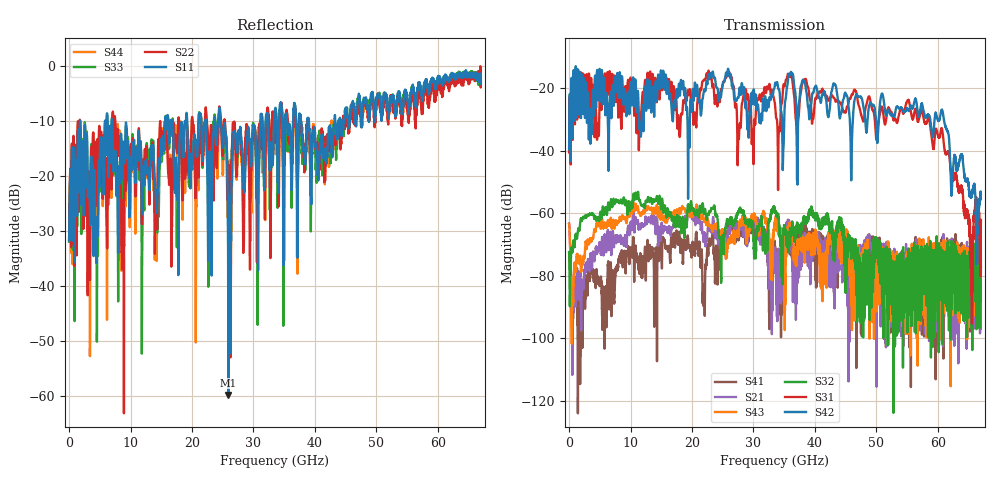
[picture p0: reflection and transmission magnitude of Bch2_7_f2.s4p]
!Agilent Technologies,N5247A,US51170199,A.09.90.13
!Agilent N5247A: A.09.90.13
!Date: Thursday, October 18, 2018 10:07:24
!Correction: S11(Full 4 Port(1,2,3,4))
!S12(Full 4 Port(1,2,3,4))
!S13(Full 4 Port(1,2,3,4))
!S14(Full 4 Port(1,2,3,4))
!S21(Full 4 Port(1,2,3,4))
!S22(Full 4 Port(1,2,3,4))
!S23(Full 4 Port(1,2,3,4))
!S24(Full 4 Port(1,2,3,4))
!S31(Full 4 Port(1,2,3,4))
!S32(Full 4 Port(1,2,3,4))
!S33(Full 4 Port(1,2,3,4))
!S34(Full 4 Port(1,2,3,4))
!S41(Full 4 Port(1,2,3,4))
!S42(Full 4 Port(1,2,3,4))
!S43(Full 4 Port(1,2,3,4))
!S44(Full 4 Port(1,2,3,4))
!S4P File: Measurements: <S11,S12,S13,S14>,
!<S21,S22,S23,S24>,
!<S31,S32,S33,S34>,
!<S41,S42,S43,S44>:
# Hz S  dB  R 50
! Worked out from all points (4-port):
!   6701 points, 10 MHz to 67 GHz, reference 50 ohm
!   strongest paths, dB at 10 MHz, 16.76 GHz, 33.51 GHz, 50.25 GHz, 67 GHz:
!     S42: -39.5, -28.6, -18.4, -34.5, -54.0
!     S31: -40.5, -21.7, -25.1, -31.9, -62.1
!     S32: -72.4, -62.0, -59.2, -75.8, -79.0
!     S43: -63.3, -59.6, -62.2, -69.1, -74.9
!     S21: -63.2, -64.4, -71.0, -80.1, -83.1
!     S41: -72.7, -68.5, -71.1, -77.5, -77.2
!   lowest |S11| = -59.8 dB at 25.91 GHz (marker M1), VSWR 1.00, Z = 50 + j0.0928 ohm
!   |S11| at or under -10 dB: 7.028 GHz to 15.65 GHz (8.622 GHz wide, 76 % of centre); 24.66 GHz to 31.12 GHz (6.453 GHz wide, 23.1 % of centre); 38.98 GHz to 43.16 GHz (4.185 GHz wide, 10.2 % of centre)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
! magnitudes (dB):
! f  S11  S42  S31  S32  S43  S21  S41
! 10 MHz  -31.7  -39.5  -40.5  -72.4  -63.3  -63.2  -72.7
! 11 GHz  -15.1  -27.5  -34.4  -55.3  -58.9  -63.0  -73.9
! 24.47 GHz  -7.8  -23.1  -24.2  -67.9  -65.5  -68.9  -76.4
! 25.91 GHz  -59.8  -13.9  -15.7  -62.9  -68.9  -64.8  -64.2
! 27.66 GHz  -12.0  -21.3  -35.0  -59.1  -64.2  -64.6  -67.5
! 55.14 GHz  -7.0  -26.8  -23.7  -78.1  -74.6  -82.6  -74.6
! 67 GHz  -3.2  -54.0  -62.1  -79.0  -74.9  -83.1  -77.2
